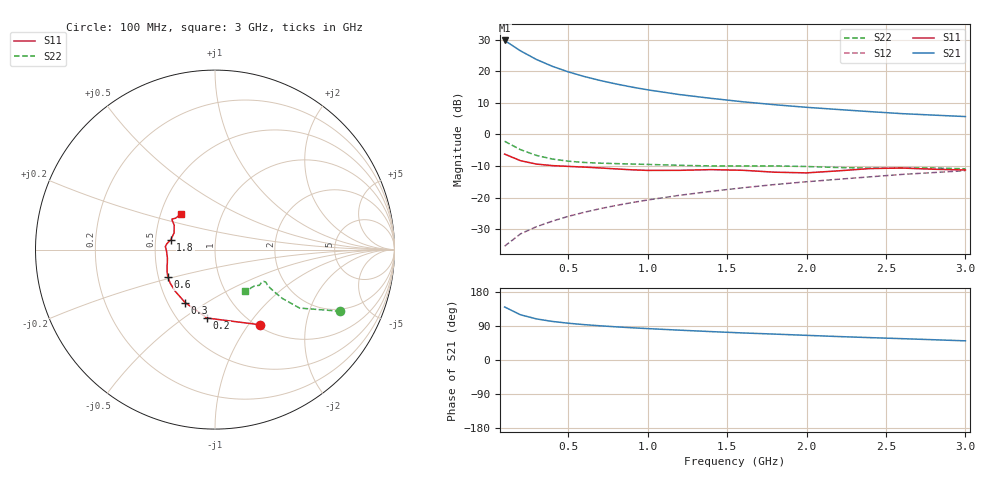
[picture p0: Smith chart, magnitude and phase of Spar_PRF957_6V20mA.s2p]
! Filename:  PRF957P.S2P  Version:  3.0
! NXP part #:  PRF957  Date:  Nov 1998
! Bias condition:  Vce=6V, Ic=20mA
#  MHz  S  MA  R 50
! Freq  S11  S21  S12  S22
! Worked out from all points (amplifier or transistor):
!   20 points, 100 MHz to 3 GHz, reference 50 ohm
!   highest |S21| = 29.7 dB at 100 MHz (marker M1)
!   |S21| within 3 dB of that: start of sweep to 191.3 MHz
!   unconditionally stable (mu >= 1): 823.2 MHz to end of sweep
!   at 400 MHz: K = 0.87, MSG = 24.5 dB, |S12| = -27.5 dB
!   at 1.2 GHz: K = 1.04, MAG = 14.8 dB, |S12| = -19.3 dB
!   at 3 GHz: K = 1.03, MAG = 7.5 dB, |S12| = -11.5 dB
!   lowest NFmin = 1.59 dB at 500 MHz
!   S11 on the Smith chart (normalised r, x): 100 MHz: 1.03, -1.14; 200 MHz: 0.69, -0.62; 300 MHz: 0.61, -0.41; 600 MHz: 0.56, -0.19; 1.8 GHz: 0.60, +0.07; 3 GHz: 0.64, +0.27
100  0.4881 -59.1  30.64 139.9  0.01706 69.5  0.7789 -26.2
200  0.3839 -96.4  20.98 119.3  0.02671 65.5  0.5731 -34.6
300  0.3392 -119.2  15.33 108.5  0.03463 66.7  0.4652 -35.9
400  0.321 -133.7  11.96 101.8  0.04239 68.8  0.408 -35.5
500  0.312 -143.1  9.77 97.0  0.05046 70.7  0.3771 -34.9
600  0.304 -149.7  8.256 93.3  0.05851 72.0  0.36 -34.4
700  0.2947 -154.9  7.142 90.3  0.06674 73.2  0.3507 -33.9
800  0.2847 -159.8  6.294 87.6  0.07498 74.0  0.3452 -33.4
900  0.2754 -164.7  5.614 85.1  0.08331 74.7  0.3402 -32.9
1000  0.2695 -169.7  5.074 82.9  0.09173 75.1  0.3353 -32.6
1200  0.2702 -178.4  4.272 78.7  0.1087 75.4  0.3244 -33.1
1400  0.2771 176.4  3.718 74.9  0.1257 75.4  0.3174 -35.3
1600  0.2705 173.2  3.282 71.4  0.1432 75.2  0.3172 -37.6
1800  0.2524 167.4  2.946 68.3  0.161 74.8  0.3171 -38.9
2000  0.2463 157.6  2.683 65.1  0.1782 74.4  0.3105 -40.1
2200  0.2651 149.1  2.476 61.9  0.1952 73.9  0.2992 -42.6
2400  0.2881 145.8  2.291 59.0  0.2132 73.0  0.2928 -46.5
2600  0.2938 144.7  2.131 56.3  0.2328 72.1  0.2941 -50.0
2800  0.2811 141.5  2.019 53.5  0.249 71.5  0.2939 -52.1
3000  0.2734 133.8  1.915 50.6  0.2667 71.0  0.2858 -54.0
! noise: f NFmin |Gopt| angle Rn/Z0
500  1.59  0.02  146  0.18
800  1.76  0.14  116  0.19
900  1.92  0.17  126  0.13
1000  1.92  0.16  109  0.22
1500  1.85  0.39  133  0.1
2000  2.22  0.31  -149  0.18
